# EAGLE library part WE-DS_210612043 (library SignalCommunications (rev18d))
WE-DS D-SUB-Filter Connectors Bent 90° Characteristics Standard type filtered with 1000 pF High attenuation of more than 40 dB @ 180 MHz Choice of earthing metal sheet or high speed earthing clip Rated voltage: 100 VDC Rated current @ 20 ºC: 5 A Withstand voltage: 250 VRMS Insulation resistance: min. 1000 MΩ Operating temperature: –55 ºC to +125 ºC Applications Filtering of interfaces External connection to -printer -sensor -display Details see: http://katalog.we-online.de/en/pbs/Filter_abgewinkelt Created on 2015-05-04 2015 (C) Wurth Elektronik
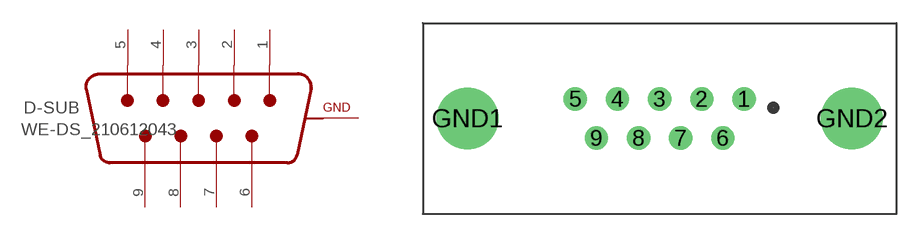
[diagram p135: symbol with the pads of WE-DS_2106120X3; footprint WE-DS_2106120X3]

Designator prefix D-SUB

## WE-DS_210612043 (WE-NUMBER: 210612043/9pins_female)  [WE-DS_2106120X3]
1  5  pas
2  4  pas
3  3  pas
4  2  pas
5  1  pas
6  9  pas
7  8  pas
8  7  pas
9  6  pas
GND1  GND  pwr
GND2  GND  pwr

## Footprint WE-DS_2106120X3 (pad centres in mm)
drill 1: 1 5.49,1.27; 2 2.74,1.27; 3 0,1.27; 4 -2.74,1.27; 5 -5.49,1.27; 6 4.11,-1.27; 7 1.37,-1.27; 8 -1.37,-1.27; 9 -4.11,-1.27
drill 3: GND1 -12.5,0; GND2 12.5,0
